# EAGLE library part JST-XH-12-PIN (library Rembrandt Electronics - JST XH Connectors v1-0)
JST XH Connector 2 Pin Wire to board connector. Pitch: 2,54 mm, (0.100") Number of pins: 12 Created by Rembrandt Electronics www.rembrandtelectronics.com
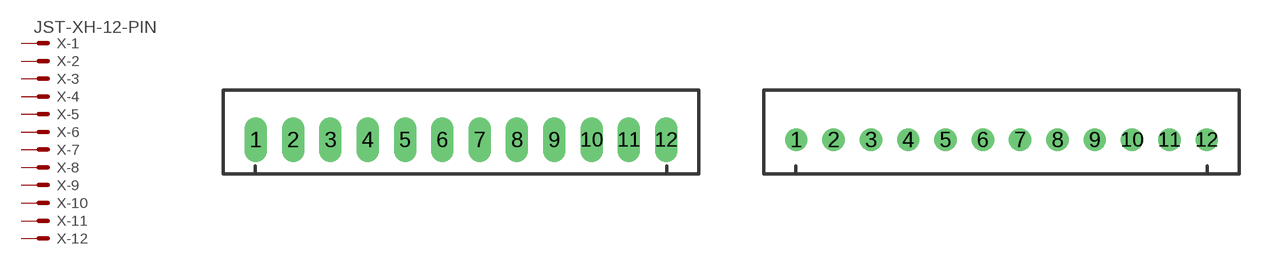
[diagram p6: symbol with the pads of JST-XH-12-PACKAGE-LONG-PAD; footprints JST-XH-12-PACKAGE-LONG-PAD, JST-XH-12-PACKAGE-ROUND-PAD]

Designator prefix X; gates -1=MV -2=M -3=M -4=M -5=M -6=M -7=M -8=M -9=M -10=M -11=M -12=M

## JST-XH-12-PIN-LONG-PAD  [JST-XH-12-PACKAGE-LONG-PAD]
1  -1:S  pas
2  -2:S  pas
3  -3:S  pas
4  -4:S  pas
5  -5:S  pas
6  -6:S  pas
7  -7:S  pas
8  -8:S  pas
9  -9:S  pas
10  -10:S  pas
11  -11:S  pas
12  -12:S  pas

## JST-XH-12-PIN-ROUND-PAD  [JST-XH-12-PACKAGE-ROUND-PAD]
Pads as for JST-XH-12-PACKAGE-LONG-PAD

## Footprint JST-XH-12-PACKAGE-LONG-PAD (pad centres in mm)
JST XH Connector Long Pads (Package) Wire to board connector. Pitch: 2,54 mm, (0.100") Number of pins: 12 Created by Rembrandt Electronics www.rembrandtelectronics.com
drill 1.016 long: 1 -13.97,0; 2 -11.43,0; 3 -8.89,0; 4 -6.35,0; 5 -3.81,0; 6 -1.27,0; 7 1.27,0; 8 3.81,0; 9 6.35,0; 10 8.89,0; 11 11.43,0; 12 13.97,0

## Footprint JST-XH-12-PACKAGE-ROUND-PAD (pad centres in mm)
JST XH Connector Round Pads (Package) Wire to board connector. Pitch: 2,54 mm, (0.100") Number of pins: 12 Created by Rembrandt Electronics www.rembrandtelectronics.com
drill 1.016: 1 -13.97,0; 2 -11.43,0; 3 -8.89,0; 4 -6.35,0; 5 -3.81,0; 6 -1.27,0; 7 1.27,0; 8 3.81,0; 9 6.35,0; 10 8.89,0; 11 11.43,0; 12 13.97,0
